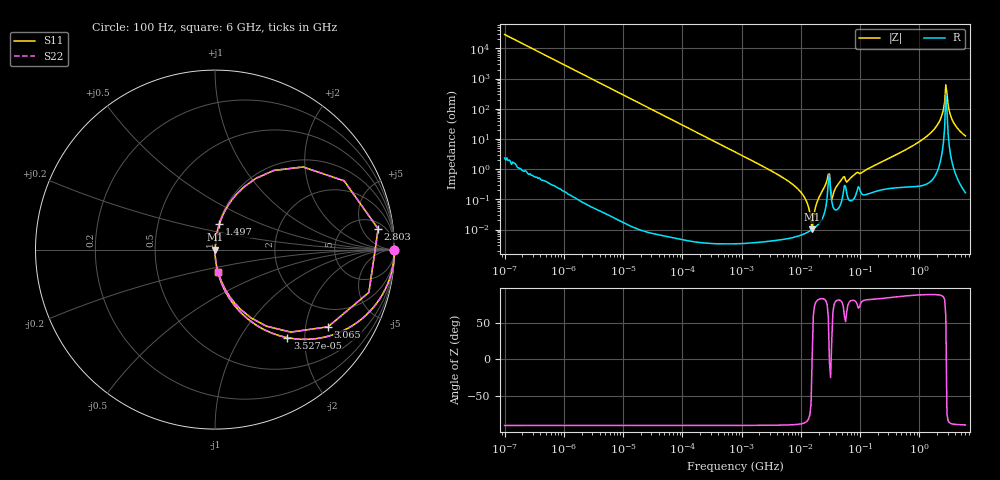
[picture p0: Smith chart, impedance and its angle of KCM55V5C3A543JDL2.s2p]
!Murata Part Number: KCM55V5C3A543JDL2
!These Parameters are Measured in Series Mode Connection
!Data Generated on Mar 13, 2026
!  o--ll--o
!Port1  Port2
!  o------o
!Operation Temp=25[degC], DC Bias Voltage=0[V]
!Freq. Start=100[Hz] Stop=6[GHz] 401[Steps]
# Hz S RI R 50
!Freq.(Hz) S11(Real) S11(Imag) S21(Real) S21(Imag) S12(Real) S12(Imag) S22(Real) S22(Imag)
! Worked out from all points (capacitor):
!   401 points, 100 Hz to 6 GHz, reference 50 ohm
!   read as one part in series: C = 54.9 nF near 109 Hz
!   lowest |Z| = 10.1 mohm at 15.56 MHz (marker M1)
!   series resonance near 15.53 MHz, so ESL is about 1.9 nH
!   S11 on the Smith chart (normalised r, x): 100 Hz: open; 35.27 kHz: 1.00, -1.64; 1.497 GHz: 1.01, +0.30; 2.803 GHz: 7, +11; 3.065 GHz: 1.30, -2.67; 6 GHz: 1.00, -0.25
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100  1 -0.00345  1.22e-05 0.00345  1.22e-05 0.00345  1 -0.00345
2008  0.9952 -0.069  0.00479 0.069  0.00479 0.069  0.9952 -0.069
10527  0.8833 -0.321  0.1167 0.321  0.1167 0.321  0.8833 -0.321
35265  0.4029 -0.4904  0.5971 0.4904  0.5971 0.4904  0.4029 -0.4904
40335  0.3402 -0.4737  0.6598 0.4737  0.6598 0.4737  0.3402 -0.4737
112960  0.0617 -0.2406  0.9383 0.2406  0.9383 0.2406  0.0617 -0.2406
774597  0.00142 -0.0373  0.9986 0.0373  0.9986 0.0373  0.00142 -0.0373
7947587  6.37e-05 -0.00272  0.9999 0.00272  0.9999 0.00272  6.37e-05 -0.00272
1.189169e7  7.56e-05 -0.00104  0.9999 0.00104  0.9999 0.00104  7.56e-05 -0.00104
1.555665e7  0.0001 6.7e-06  0.9999 -6.7e-06  0.9999 -6.7e-06  0.0001 6.7e-06
2.784235e7  0.00118 0.00431  0.9988 -0.00431  0.9988 -0.00431  0.00118 0.00431
3.482834e7  0.000575 0.0012  0.9994 -0.0012  0.9994 -0.0012  0.000575 0.0012
4.983056e7  0.00104 0.00464  0.999 -0.00464  0.999 -0.00464  0.00104 0.00464
3.124326e8  0.0028 0.0229  0.9972 -0.0229  0.9972 -0.0229  0.0028 0.0229
1.497423e9  0.0248 0.1436  0.9752 -0.1436  0.9752 -0.1436  0.0248 0.1436
2.048624e9  0.092 0.2743  0.908 -0.2743  0.908 -0.2743  0.092 0.2743
2.450438e9  0.3276 0.441  0.6724 -0.441  0.6724 -0.441  0.3276 0.441
2.802721e9  0.9091 0.1155  0.0909 -0.1155  0.0909 -0.1155  0.9091 0.1155
3.065283e9  0.6297 -0.4301  0.3703 0.4301  0.3703 0.4301  0.6297 -0.4301
3.352442e9  0.2851 -0.4261  0.7149 0.4261  0.7149 0.4261  0.2851 -0.4261
3.8344e9  0.109 -0.2971  0.891 0.2971  0.891 0.2971  0.109 -0.2971
6e9  0.0171 -0.1232  0.9829 0.1232  0.9829 0.1232  0.0171 -0.1232
